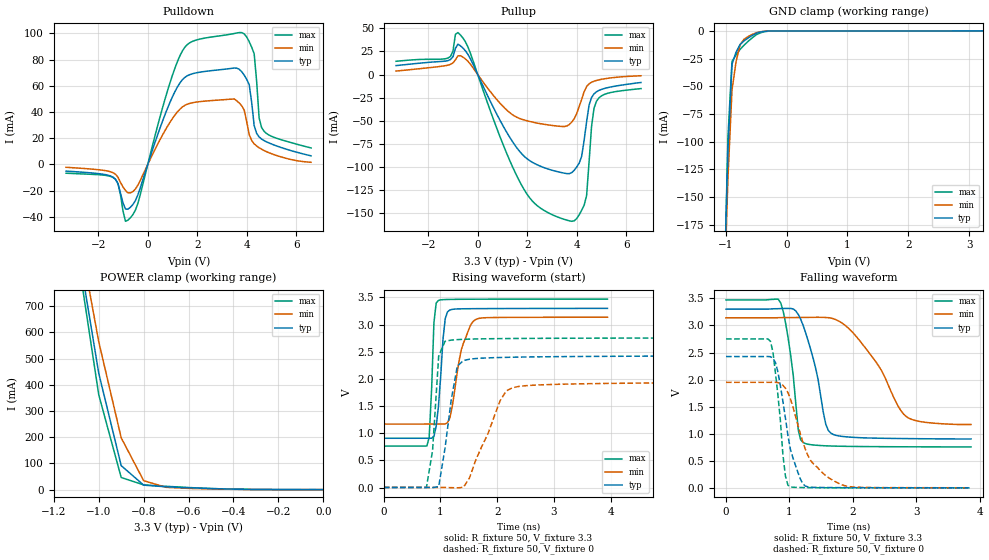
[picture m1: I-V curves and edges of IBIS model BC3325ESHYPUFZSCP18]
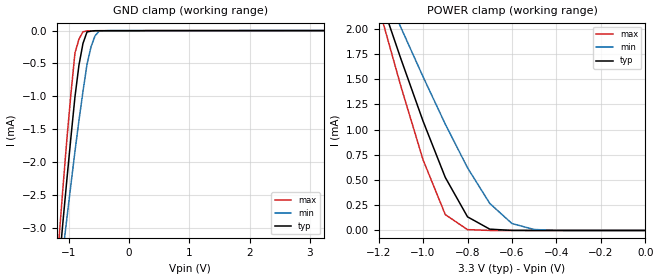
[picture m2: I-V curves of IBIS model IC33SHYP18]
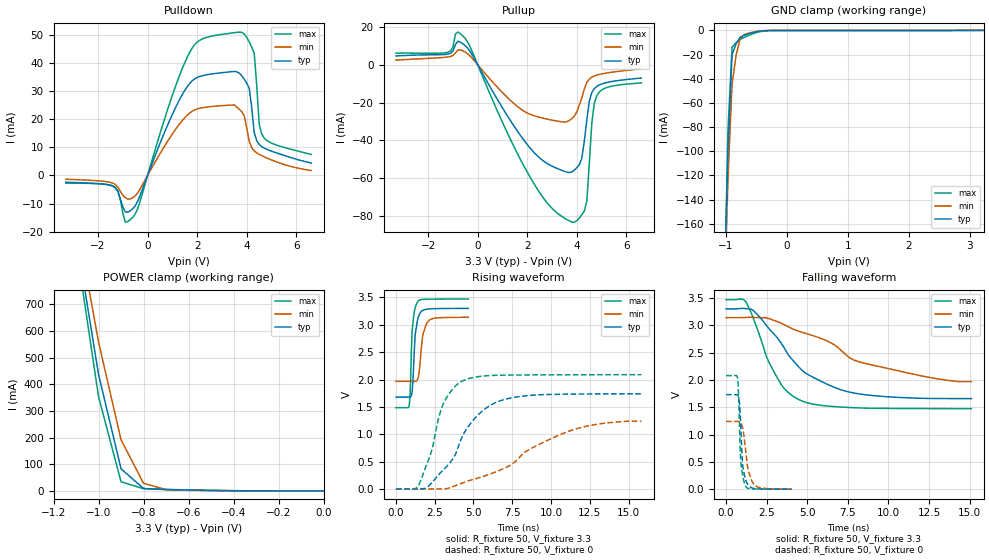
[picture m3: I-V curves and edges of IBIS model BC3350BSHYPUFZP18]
| TEXAS INSTRUMENTS INCORPORATED
| Standard Linear and Logic Group
| IBIS Model of TLK100
[IBIS Ver]   3.2
[Comment char]  |_char
[File Name]   tlk100.ibs
[File Rev]   1.0 | b_die
[Date]   June 17, 2009
[Source]   Data created from TI-SPICE simulations at TI-SLL.
[Notes]   The following is an IBIS list for tlk100 PG1.
   All NON Digital I/O's are referenced in the pin list section as NC
[Disclaimer] Property of Texas Instruments Incorporated.  Unauthorized
  reproduction and/or distribution is strictly prohibited.
  This product is protected under copyright law.
  Created  2008, (C) Copyright  2008, Texas Instruments
  Incorporated, All Rights Reserved
  UNLESS THERE IS A SIGNED, WRITTEN AGREEMENT TO THE
  CONTRARY, TEXAS INSTRUMENTS (TI) IS PROVIDING THE IBIS
  MODELS  AND WITHOUT ANY WARRANTY, EXPRESSED OR
  IMPLIED.  TI assumes no liability for:
   1) the accuracy of the IBIS models provided to your
   company;
   2) the proper functioning of these IBIS Models in your
   design or for any resulting applications; or
   3) infringement of patents, copyrights or intellectual
   property rights resulting from your use of these IBIS
   models.
  TI provides IBIS Models as a service to our customers.
  You and your company shall not distribute, sell or give
  these models to anyone else without prior written
  permission from TI.
  TI reserves the right to make changes to our products or
  to discontinue any semiconductor product or service
  without notice, and advises our customers to obtain the
  latest version of relevant information to verify, before
  placing orders, that the information being relied on is
  current.
  Please be aware that your receipt and use of the IBIS
  information provided shall serve as acceptance of these
  terms and conditions.  If you do not accept these terms,
  you should return or destroy the IBIS models and any
  other accompanying information immediately.
[Component]   TLK100
[Manufacturer]   Texas Instruments, Inc.
[Package]
|   typ   min   max
R_pkg   0.1808556   0.15587   0.20997
L_pkg   2.067785n   1.73999n   2.47426n
C_pkg   0.359423p   0.31402p   0.40767p
[Pin]   signal_name   model_name   R_pin   L_pin   C_pin
1   VA11_PFBIN1   NC   0.19904 2.29852n 0.39263p
2   V18_PFBIN1   NC   0.18877 2.139n   0.40767p
3   RBIAS   NC   0.17948 2.0244n  0.37601p
4   V18_PFBIN2   NC   0.17152 1.9359n  0.35636p
5   XFMRM_B   NC   0.16678 1.89815n 0.35587p
6   XFMRP_B   NC   0.16617 1.89788n 0.34747p
7   VA11_PFBIN2   NC   0.16834 1.93016n 0.34201p
8   XFMRM_A   NC   0.1744  2.01382n 0.36129p
9   XFMRP_A   NC   0.18359 2.11817n 0.38275p
10   VA11_PFOUT   NC   0.19428 2.24924n 0.38613p
11   VDD33_VA11   POWER   0.19969 2.30792n 0.38851p
12   CLK25OUT   OC3350BSFZP18   0.20538 2.4046n  0.37478p
13   TXD_0   BC3350BSHYPDFZP18   0.20997 2.47426n 0.38697p
14   TXD_1   IC33SHYPDFZP18   0.19966 2.3091n  0.39801p
15   TXD_2   IC33SHYPDFZP18   0.1889  2.17117n 0.37745p
16   TXD_3   IC33SHYPDFZP18   0.18098 2.08172n 0.3692p
17   VDD33_IO   POWER   0.17615 2.04242n 0.361p
18   TX_EN   BC3350BSHYPDFZP18   0.17569 2.04377n 0.33735p
19   TX_CLK   BC3350BSHYPDFZP18   0.17809 2.0787n  0.33532p
20   VD11_PFOUT   NC   0.18301 2.14475n 0.34454p
21   VDD33_VD11   POWER   0.18719 2.17402n 0.34929p
22   CRS   BC3350BSHYPUFZP18   0.18861 2.16682n 0.36646p
23   RX_CLK   OC3350BSFZP18   0.19774 2.28065n 0.38922p
24   COL   BC3350BSHYPUFZP18   0.20769 2.44028n 0.36199p
25   RXD_0   BC3350BSHYPDFZP18   0.20331 2.37343n 0.35906p
26   RXD_1   BC3350BSHYPDFZP18   0.19219 2.19592n 0.38503p
27   RXD_2   BC3350BSHYPDFZP18   0.18188 2.06395n 0.36184p
28   RXD_3   BC3350BSHYPDFZP18   0.17357 1.96837n 0.34862p
29   VDD33_IO   POWER   0.16805 1.91817n 0.34931p
30   RX_DV   BC3350BSHYPDFZP18   0.16551 1.88795n 0.32653p
31   RX_ERR   BC3350BSHYPUFZP18   0.1666  1.9028n  0.32359p
32   MDC   IC33SHYP18   0.17038 1.95113n 0.34065p
33   MDIO   BC3350CSHYFZP18   0.17963 2.05484n 0.35032p
34   LED_ACT   BC3325ESHYPUFZSCP18   0.17839 2.00872n 0.354p
35   LED_SPEED   BC3325ESHYPUFZSCP18   0.18714 2.11609n 0.37799p
36   LED_LINK   BC3325ESHYPUFZSCP18   0.19675 2.2695n  0.36477p
37   XO   NC   0.19312 2.21485n 0.36619p
38   VSS   GND   0.18201 2.03746n 0.38002p
39   XI   NC   0.17023 1.88472n 0.35463p
40   V18_PFOUT   NC   0.16204 1.79149n 0.32854p
41   VDD33_V18   POWER   0.15822 1.76741n 0.31793p
42   PWRDNN   BC3350BSHYPUFZP18   0.15804 1.77262n 0.31402p
43   RESETN   IC33SHYPUFZP18   0.15587 1.73999n 0.31695p
44   TCK   IC33SHYPUFZP18   0.15704 1.74986n 0.33687p
45   TDI   IC33SHYPUFZP18   0.16188 1.78902n 0.33864p
46   TMS   IC33SHYPUFZP18   0.17074 1.89173n 0.35843p
47   TDO   OC3350BSFZP18   0.18273 2.04732n 0.3813p
48   TRSTN   IC33SHYPUFZP18   0.19463 2.23092n 0.36879p
49   VSS   GND   0.00067 0.00868n 2.08228p
| Models and submodels in the file (8): BC3325ESHYPUFZSCP18 (I/O), IC33SHYP18 (Input), BC3350BSHYPUFZP18 (I/O), BC3350BSHYPDFZP18 (I/O), IC33SHYPDFZP18 (Input), IC33SHYPUFZP18 (Input), OC3350BSFZP18 (I/O), BC3350CSHYFZP18 (I/O)
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|   Model Cell BC3325ESHYPUFZSCP18
[Model]   BC3325ESHYPUFZSCP18
Model_type   I/O
Polarity   Non-Inverting
Enable   Active-Low
Vinl =  0.8V
Vinh =  2V
Cref =  15.0000pF
Rref =  100.0000M
Vref =  0V
Vmeas =  1.65
C_comp   2.566034p   2.494321p   2.623693p
[Model Spec]
Vinl   0.8V   0.8V   0.8V
Vinh   2V   2V   2V
[Temperature Range]   25   125   -40
[Voltage Range]   3.3   3.14   3.47
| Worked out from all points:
|   slope of the pulldown table from 0 to 0.495 V, typ, clamps not added: 17.8 ohm
|   slope of the pullup table from 0 to 0.495 V, typ, clamps not added: 17.6 ohm
|   GND clamp passes 1 mA (typ) near -0.42 V on its own axis
|   POWER clamp passes 1 mA (typ) near -0.34 V on its own axis
|   rising waveform, R_fixture 50, V_fixture 3.3: 20-80 % time 101ps typ, 220ps min, 61.9ps max; typ from 0.907 V to 3.3 V
|   rising waveform, R_fixture 50, V_fixture 0: 20-80 % time 203ps typ, 454ps min, 115ps max; typ from 0.002 V to 2.43 V
|   falling waveform, R_fixture 50, V_fixture 3.3: 20-80 % time 269ps typ, 600ps min, 165ps max; typ from 3.3 V to 0.905 V
|   falling waveform, R_fixture 50, V_fixture 0: 20-80 % time 226ps typ, 390ps min, 132ps max; typ from 2.42 V to 0.003 V
[POWER_clamp]
|   voltage   I(typ)   I(min)   I(max)
-3.3V     15.08A     13.67A     16.19A
-1.067V   791.8mA    876.7mA    739.7mA
-1.033V   617.9mA    720.5mA    550.8mA
-1V       444mA      564.3mA    361.9mA
-900mV    91.5mA     197.6mA    46.16mA
-800mV    17.11mA    33.99mA    18mA
-700mV    10.63mA    8.68mA     12.59mA
-400mV    1.748mA    1.071mA    1.568mA
-11.55fV  124.3nA    283.1nA    244.6nA
[Pulldown]
|   voltage   I(typ)   I(min)   I(max)
-3.3V     -5.059mA   -2.155mA   -6.66mA
-1.4V     -9.748mA   -6.303mA   -9.905mA
-800mV    -34.11mA   -21.63mA   -42.45mA
-400mV    -23.24mA   -15.83mA   -29.78mA
700mV     38.17mA    25.94mA    50mA
1.4V      64.67mA    43.88mA    86.65mA
3.7V      72.59mA    46.86mA    100.7mA
4.1V      60.89mA    22.84mA    93.69mA
4.3V      29.74mA    15.79mA    84.53mA
4.5V      21.02mA    12.79mA    35.5mA
4.6V      19.41mA    11.66mA    28.23mA
6.6V      6.581mA    1.677mA    12.61mA
[Pullup]
|   voltage   I(typ)   I(min)   I(max)
-3.3V     9.651mA    3.755mA    14.31mA
-1.2V     15.05mA    10.14mA    17.8mA
-800mV    32.8mA     20.21mA    45.37mA
-400mV    22mA       14.46mA    30.15mA
1V        -54.37mA   -33.86mA   -73.98mA
1.9V      -88.97mA   -49.34mA   -125.5mA
3.8V      -106.1mA   -51.52mA   -158.7mA
4.2V      -88.49mA   -27.05mA   -146.8mA
4.4V      -51.11mA   -13.02mA   -131mA
4.6V      -24.86mA   -8.372mA   -56.19mA
4.8V      -18.68mA   -6.397mA   -28.85mA
6.6V      -8.617mA   -1.357mA   -15.22mA
[GND_clamp]
|   voltage   I(typ)   I(min)   I(max)
-3.3V     -17.31A    -15.67A    -18.52A
-1.033V   -242.5mA   -247.9mA   -249.2mA
-966.7mV  -107.7mA   -133.3mA   -96.21mA
-900mV    -30.23mA   -53.64mA   -27.71mA
-833.3mV  -19.36mA   -27.93mA   -21.66mA
-766.7mV  -12.28mA   -12.57mA   -16.71mA
-700mV    -9.011mA   -7.551mA   -12.86mA
-566.7mV  -4.137mA   -3.208mA   -6.295mA
-500mV    -2.163mA   -1.683mA   -3.503mA
-433.3mV  -1.112mA   -895.4uA   -1.851mA
-300mV    -188.2uA   -143uA     -305.2uA
3.233V    -8.744uA   11.87uA    -45.21uA
[Ramp]
| variable   typ   min   max
dV/dt_f   1.450776/0.27124n   1.211798/0.6135665n   1.638368/0.1633701n
dV/dt_r   1.462664/0.1781939n   1.183254/0.4581737n   1.655056/98.72251p
R_load = 50
[Rising Waveform]
R_fixture = 50
V_fixture = 3.3
V_fixture_min = 3.14
V_fixture_max = 3.47
|   time   V(typ)   V(min)   V(max)
0s        907.1mV    1.168V     762.9mV
760ps     907.3mV    1.169V     766.1mV
800ps     907.3mV    1.169V     920.6mV
884ps     942.4mV    1.169V     3.034V
964ps     1.496V     1.169V     3.445V
1.084ns   3.113V     1.172V     3.463V
1.164ns   3.27V      1.277V     3.465V
1.368ns   3.292V     2.542V     3.467V
1.608ns   3.294V     3.088V     3.469V
3.944ns   3.299V     3.137V     3.47V
[Rising Waveform]
R_fixture = 50
V_fixture = 0
V_fixture_min = 0
V_fixture_max = 0
|   time   V(typ)   V(min)   V(max)
0s        1.739mV    1.142mV    2.323mV
752ps     1.714mV    1.145mV    730.9uV
860ps     -1.224mV   1.145mV    680.7mV
968ps     16.34mV    1.144mV    2.422V
1.08ns    726.4mV    114.5uV    2.694V
1.296ns   2.236V     -6.46mV    2.724V
1.512ns   2.363V     178.1mV    2.733V
2.052ns   2.395V     1.601V     2.743V
2.376ns   2.402V     1.861V     2.745V
10.6ns    2.428V     1.947V     2.757V
[Falling Waveform]
R_fixture = 50
V_fixture = 3.3
V_fixture_min = 3.14
V_fixture_max = 3.47
|   time   V(typ)   V(min)   V(max)
0s        3.3V       3.14V      3.47V
864ps     3.311V     3.144V     3.411V
1.02ns    3.313V     3.145V     2.442V
1.14ns    3.2V       3.147V     1.061V
1.216ns   2.998V     3.147V     837.2mV
1.572ns   1.178V     3.146V     778.2mV
1.652ns   1.012V     3.136V     774.7mV
2.28ns    921.8mV    2.456V     763.7mV
2.832ns   911.8mV    1.325V     760.2mV
3.86ns    904.7mV    1.172V     757.9mV
[Falling Waveform]
R_fixture = 50
V_fixture = 0
V_fixture_min = 0
V_fixture_max = 0
|   time   V(typ)   V(min)   V(max)
0s        2.425V     1.95V      2.751V
700ps     2.423V     1.95V      2.708V
740ps     2.395V     1.951V     2.506V
816ps     2.151V     1.945V     1.737V
936ps     1.291V     1.842V     222.2mV
1.012ns   727.8mV    1.654V     21.93mV
1.208ns   81.91mV    858.1mV    7.931mV
1.328ns   15.28mV    516.5mV    6.256mV
1.756ns   6.84mV     96.85mV    3.69mV
3.836ns   2.752mV    4.289mV    2.303mV
|   Model Cell IC33SHYP18
[Model]   IC33SHYP18
Model_type   Input
Polarity   Non-Inverting
Vinl =  0.8V
Vinh =  2V
C_comp   0.7465841p   0.6831479p   0.8220855p
[Model Spec]
Vinl   0.8V   0.8V   0.8V
Vinh   2V   2V   2V
[Temperature Range]   25   125   -40
[Voltage Range]   3.3   2.97   3.63
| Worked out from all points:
|   GND clamp passes 1 mA (typ) near -0.90 V on its own axis
|   POWER clamp passes 1 mA (typ) near -0.98 V on its own axis
[POWER_clamp]
|   voltage   I(typ)   I(min)   I(max)
-3.3V     16.09mA    13.32mA    18.73mA
-1.2V     2.351mA    2.516mA    2.221mA
-1.167V   2.136mA    2.349mA    1.958mA
-1.133V   1.92mA     2.182mA    1.695mA
-1.1V     1.705mA    2.015mA    1.432mA
-1V       1.085mA    1.525mA    701.3uA
-900mV    526.2uA    1.055mA    157.4uA
-800mV    135.4uA    621.8uA    8.521uA
-700mV    13.19uA    268.3uA    565.5nA
-600mV    617.4nA    68.7uA     453.6nA
-500mV    119.1nA    9.616uA    441.5nA
-11.55fV  95.16nA    58.97nA    392nA
[GND_clamp]
|   voltage   I(typ)   I(min)   I(max)
-3.3V     -25.77mA   -21.29mA   -28.7mA
-1.167V   -3.595mA   -3.893mA   -3.188mA
-1.1V     -2.914mA   -3.365mA   -2.395mA
-1.033V   -2.256mA   -2.848mA   -1.643mA
-900mV    -1.008mA   -1.837mA   -339.5uA
-833.3mV  -523.5uA   -1.365mA   -129.1uA
-766.7mV  -194.5uA   -923.8uA   -17.39uA
-700mV    -20.9uA    -513.1uA   -4.234uA
-633.3mV  -8.234uA   -247.5uA   -3.824uA
-566.7mV  -1.665uA   -79.74uA   -3.619uA
-500mV    -1.19uA    -9.867uA   -3.619uA
3.233V    93.9nA     106.2nA    357.7nA
|   Model Cell BC3350BSHYPUFZP18
[Model]   BC3350BSHYPUFZP18
Model_type   I/O
Polarity   Non-Inverting
Enable   Active-Low
Vinl =  0.8V
Vinh =  2V
Cref =  15.0000pF
Rref =  100.0000M
Vref =  0V
Vmeas =  1.65
C_comp   1.727272p   1.679637p   1.767235p
[Model Spec]
Vinl   0.8V   0.8V   0.8V
Vinh   2V   2V   2V
[Temperature Range]   25   125   -40
[Voltage Range]   3.3   3.14   3.47
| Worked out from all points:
|   slope of the pulldown table from 0 to 0.495 V, typ, clamps not added: 44 ohm
|   slope of the pullup table from 0 to 0.495 V, typ, clamps not added: 42.8 ohm
|   GND clamp passes 1 mA (typ) near -0.48 V on its own axis
|   POWER clamp passes 1 mA (typ) near -0.41 V on its own axis
|   rising waveform, R_fixture 50, V_fixture 3.3: 20-80 % time 226ps typ, 308ps min, 183ps max; typ from 1.68 V to 3.3 V
|   rising waveform, R_fixture 50, V_fixture 0: 20-80 % time 2.39ns typ, 4.75ns min, 1.32ns max; typ from 0.003 V to 1.74 V
|   falling waveform, R_fixture 50, V_fixture 3.3: 20-80 % time 3.22ns typ, 5.72ns min, 1.75ns max; typ from 3.3 V to 1.66 V
|   falling waveform, R_fixture 50, V_fixture 0: 20-80 % time 203ps typ, 373ps min, 161ps max; typ from 1.73 V to 0.004 V
[POWER_clamp]
|   voltage   I(typ)   I(min)   I(max)
-3.3V     15.06A     13.65A     16.18A
-1.067V   785.8mA    871.3mA    732.8mA
-1.033V   611.7mA    715.2mA    543.5mA
-1V       437.6mA    559.1mA    354.2mA
-900mV    83.18mA    192.2mA    34.46mA
-800mV    9.152mA    28.75mA    8.178mA
-700mV    4.876mA    4.858mA    5.74mA
-400mV    907.2uA    556.2uA    845.5uA
-11.55fV  111.6nA    200.9nA    235nA
[Pulldown]
|   voltage   I(typ)   I(min)   I(max)
-3.3V     -2.42mA    -1.355mA   -2.742mA
-1.4V     -3.866mA   -2.765mA   -3.735mA
-900mV    -12.98mA   -7.875mA   -16.63mA
-700mV    -12.58mA   -8.35mA    -15.75mA
1.7V      32.7mA     22.18mA    43.75mA
3.6V      36.79mA    24.24mA    50.83mA
3.9V      34.2mA     21.08mA    50.21mA
4.1V      30.97mA    12.06mA    47.43mA
4.3V      15.29mA    8.758mA    43.35mA
4.5V      11.02mA    7.482mA    18.29mA
4.6V      10.26mA    7.017mA    14.71mA
6.6V      4.411mA    1.71mA     7.432mA
[Pullup]
|   voltage   I(typ)   I(min)   I(max)
-3.3V     4.71mA     2.514mA    6.161mA
-1.2V     5.694mA    4.171mA    6.671mA
-1V       7.232mA    4.973mA    9.382mA
-900mV    10.66mA    6.233mA    16.33mA
-600mV    11.14mA    7.389mA    15.31mA
2.2V      -45.34mA   -26.59mA   -61.37mA
3.8V      -56.6mA    -28.41mA   -83.18mA
4.2V      -49.34mA   -17.47mA   -79.29mA
4.4V      -29.22mA   -9.297mA   -72.12mA
4.6V      -14.75mA   -6.534mA   -31.03mA
4.8V      -11.42mA   -5.437mA   -16.4mA
6.6V      -6.969mA   -2.118mA   -9.572mA
[GND_clamp]
|   voltage   I(typ)   I(min)   I(max)
-3.3V     -17.3A     -15.65A    -18.51A
-1.033V   -232.2mA   -237.1mA   -236.8mA
-966.7mV  -97.17mA   -123.1mA   -82.58mA
-900mV    -20.21mA   -44.63mA   -13.94mA
-833.3mV  -11mA      -20.53mA   -10.18mA
-766.7mV  -5.632mA   -6.818mA   -7.479mA
-700mV    -4.109mA   -3.501mA   -5.844mA
-500mV    -1.141mA   -861.8uA   -1.82mA
-300mV    -166.1uA   -110.3uA   -270.5uA
3.233V    -8.733uA   10uA       -45.21uA
[Ramp]
| variable   typ   min   max
dV/dt_f  0.9915771/3.236911n   0.7637923/6.725215n   1.205268/1.748241n
dV/dt_r   1.046581/2.405104n   0.7678008/4.959754n   1.253757/1.326356n
R_load = 50
[Rising Waveform]
R_fixture = 50
V_fixture = 3.3
V_fixture_min = 3.14
V_fixture_max = 3.47
|   time   V(typ)   V(min)   V(max)
0s        1.68V      1.967V     1.487V
852ps     1.68V      1.968V     1.515V
900ps     1.681V     1.968V     1.648V
1.044ns   1.771V     1.968V     2.883V
1.236ns   2.8V       1.968V     3.302V
1.376ns   3.06V      1.989V     3.408V
1.52ns    3.195V     2.191V     3.451V
1.76ns    3.266V     2.842V     3.464V
2.092ns   3.289V     3.067V     3.468V
4.668ns   3.299V     3.137V     3.47V
[Rising Waveform]
R_fixture = 50
V_fixture = 0
V_fixture_min = 0
V_fixture_max = 0
|   time   V(typ)   V(min)   V(max)
0s        3.146mV    1.893mV    4.431mV
1.452ns   4.217mV    933.1uV    59.77mV
2.26ns    98.61mV    2.873mV    657.8mV
3.068ns   355.4mV    4.373mV    1.566V
3.712ns   570.2mV    48.77mV    1.843V
4.36ns    1.007V     119.4mV    1.984V
5.652ns   1.444V     233.7mV    2.065V
7.268ns   1.655V     419.2mV    2.082V
11.31ns   1.734V     1.073V     2.088V
15.83ns   1.74V      1.24V      2.089V
[Falling Waveform]
R_fixture = 50
V_fixture = 3.3
V_fixture_min = 3.14
V_fixture_max = 3.47
|   time   V(typ)   V(min)   V(max)
0s        3.3V       3.14V      3.47V
1.228ns   3.303V     3.143V     3.429V
1.692ns   3.267V     3.144V     3.119V
2.46ns    3.006V     3.137V     2.447V
3.08ns    2.799V     3.076V     2.08V
3.696ns   2.528V     2.996V     1.808V
4.62ns    2.194V     2.879V     1.624V
6.468ns   1.891V     2.677V     1.519V
8.008ns   1.755V     2.35V      1.492V
15.11ns   1.66V      1.971V     1.477V
[Falling Waveform]
R_fixture = 50
V_fixture = 0
V_fixture_min = 0
V_fixture_max = 0
|   time   V(typ)   V(min)   V(max)
0s        1.732V     1.243V     2.081V
696ps     1.73V      1.243V     2.056V
780ps     1.676V     1.244V     1.659V
864ps     1.416V     1.231V     768.1mV
904ps     1.185V     1.218V     505.5mV
1.028ns   429.3mV    1.118V     241.7mV
1.236ns   149.4mV    635.3mV    44.53mV
1.4ns     69.06mV    312.2mV    14.04mV
1.812ns   12.91mV    65.79mV    7.243mV
4.036ns   4.391mV    5.043mV    4.639mV
